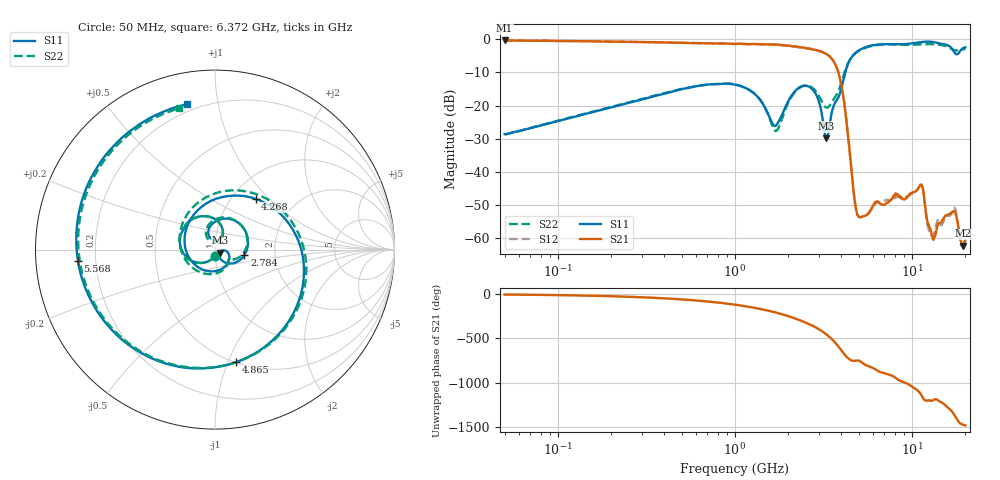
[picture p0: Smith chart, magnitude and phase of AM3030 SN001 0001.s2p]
# Hz S DB R 50
!freq MagS11 AngS11 MagS21 AngS21 MagS12 AngS12 MagS22 AngS22
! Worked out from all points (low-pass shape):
!   1601 points, 50 MHz to 20.05 GHz, reference 50 ohm
!   highest |S21| = -0.43 dB at 50 MHz (marker M1); lowest = -62.2 dB at 19.39 GHz (marker M2)
!   |S21| within 3 dB of the highest: start of sweep to 2.912 GHz
!   lowest |S11| = -29.9 dB at 3.283 GHz (marker M3), VSWR 1.07, Z = 52.8 - j1.8 ohm
!   |S11| at or under -10 dB: start of sweep to 4.204 GHz
!   |S22| runs from -28.7 to -1.5 dB; largest |S21 - S12| = 0.019
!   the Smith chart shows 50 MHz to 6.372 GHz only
!   S11 on the Smith chart (normalised r, x): 50 MHz: 1.00, -0.07; 2.784 GHz: 1.39, -0.09; 4.268 GHz: 1.28, +0.83; 4.865 GHz: 0.50, -1.07; 5.568 GHz: 0.13, -0.04; 6.372 GHz: 0.16, +0.81
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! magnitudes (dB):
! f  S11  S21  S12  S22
! 50 MHz  -28.6  -0.4  -0.5  -28.7
! 135.9 MHz  -22.8  -0.7  -0.7  -22.7
! 369.6 MHz  -16.9  -1.0  -1.0  -16.7
! 1.005 GHz  -13.7  -1.5  -1.4  -13.7
! 1.346 GHz  -17.4  -1.5  -1.6  -17.4
! 1.704 GHz  -26.0  -1.7  -1.7  -27.7
! 2.174 GHz  -15.8  -2.2  -2.3  -16.1
! 2.722 GHz  -15.0  -3.1  -3.0  -14.6
! 2.784 GHz  -15.6  -3.2  -3.0  -15.0
! 3.283 GHz  -29.9  -4.5  -4.5  -20.6
! 3.843 GHz  -17.5  -10.0  -10.1  -15.7
! 4.268 GHz  -8.8  -24.8  -24.5  -8.3
! 4.865 GHz  -3.9  -51.9  -52.0  -4.0
! 5.568 GHz  -2.3  -52.8  -53.0  -2.5
! 6.372 GHz  -1.7  -48.8  -49.0  -1.8
! 7.402 GHz  -1.5  -48.8  -48.6  -1.6
! 11.22 GHz  -0.9  -43.8  -43.6  -1.6
! 12.79 GHz  -0.8  -57.6  -58.4  -1.5
! 13.33 GHz  -1.0  -60.0  -58.7  -1.6
! 17.32 GHz  -3.8  -51.8  -50.8  -3.3
! 19.39 GHz  -2.8  -62.2  -61.9  -3.1
! 20.05 GHz  -2.5  -60.5  -59.9  -3.1
